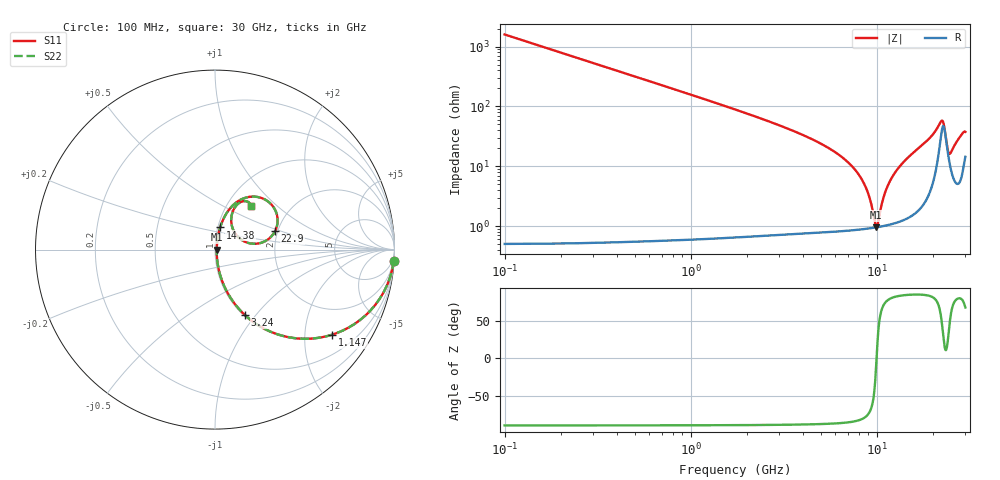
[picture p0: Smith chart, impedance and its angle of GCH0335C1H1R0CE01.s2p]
!Murata Part Number: GCH0335C1H1R0CE01
!These Parameters are Measured in Series Mode Connection
!Data Generated on Jun 19, 2026
!  o--ll--o
!Port1  Port2
!  o------o
!Operation Temp=25[degC], DC Bias Voltage=0[V]
!Freq. Start=100[MHz] Stop=30[GHz] 401[Steps]
# Hz S RI R 50
!Freq.(Hz) S11(Real) S11(Imag) S21(Real) S21(Imag) S12(Real) S12(Imag) S22(Real) S22(Imag)
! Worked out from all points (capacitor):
!   401 points, 100 MHz to 30 GHz, reference 50 ohm
!   read as one part in series: C = 1 pF near 249.5 MHz
!   lowest |Z| = 960 mohm at 9.967 GHz (marker M1)
!   series resonance near 9.992 GHz, so ESL is about 250 pH
!   S11 on the Smith chart (normalised r, x): 100 MHz: 1, -32; 1.147 GHz: 1.01, -2.74; 3.24 GHz: 1.01, -0.88; 14.38 GHz: 1.03, +0.26; 22.9 GHz: 1.94, +0.45; 30 GHz: 1.29, +0.70
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1e8  0.996 -0.0626  0.00395 0.0626  0.00395 0.0626  0.996 -0.0626
3.2425e8  0.9599 -0.1957  0.0401 0.1957  0.0401 0.1957  0.9599 -0.1957
5.485e8  0.8928 -0.3085  0.1072 0.3085  0.1072 0.3085  0.8928 -0.3085
1.1465e9  0.6516 -0.4743  0.3484 0.4743  0.3484 0.4743  0.6516 -0.4743
2.11825e9  0.3412 -0.4695  0.6588 0.4695  0.6588 0.4695  0.3412 -0.4695
3.2395e9  0.1663 -0.3643  0.8337 0.3643  0.8337 0.3643  0.1663 -0.3643
5.10825e9  0.0574 -0.2164  0.9426 0.2164  0.9426 0.2164  0.0574 -0.2164
8.3225e9  0.0122 -0.0585  0.9878 0.0585  0.9878 0.0585  0.0122 -0.0585
9.07e9  0.01 -0.031  0.99 0.031  0.99 0.031  0.01 -0.031
9.967e9  0.00947 -0.000815  0.9905 0.000815  0.9905 0.000815  0.00947 -0.000815
1.01165e10  0.00956 0.00399  0.9904 -0.00399  0.9904 -0.00399  0.00956 0.00399
1.078925e10  0.0105 0.0249  0.9895 -0.0249  0.9895 -0.0249  0.0105 0.0249
1.16115e10  0.0128 0.0491  0.9872 -0.0491  0.9872 -0.0491  0.0128 0.0491
1.437725e10  0.0287 0.1237  0.9713 -0.1237  0.9713 -0.1237  0.0287 0.1237
1.505e10  0.0345 0.141  0.9655 -0.141  0.9655 -0.141  0.0345 0.141
2.005825e10  0.1379 0.2754  0.8621 -0.2754  0.8621 -0.2754  0.1379 0.2754
2.17775e10  0.2794 0.2785  0.7206 -0.2785  0.7206 -0.2785  0.2794 0.2785
2.289875e10  0.334 0.1015  0.666 -0.1015  0.666 -0.1015  0.334 0.1015
2.424425e10  0.1388 0.061  0.8612 -0.061  0.8612 -0.061  0.1388 0.061
2.50665e10  0.0974 0.1206  0.9026 -0.1206  0.9026 -0.1206  0.0974 0.1206
2.768275e10  0.1159 0.2422  0.8841 -0.2422  0.8841 -0.2422  0.1159 0.2422
3e10  0.1998 0.2431  0.8002 -0.2431  0.8002 -0.2431  0.1998 0.2431
